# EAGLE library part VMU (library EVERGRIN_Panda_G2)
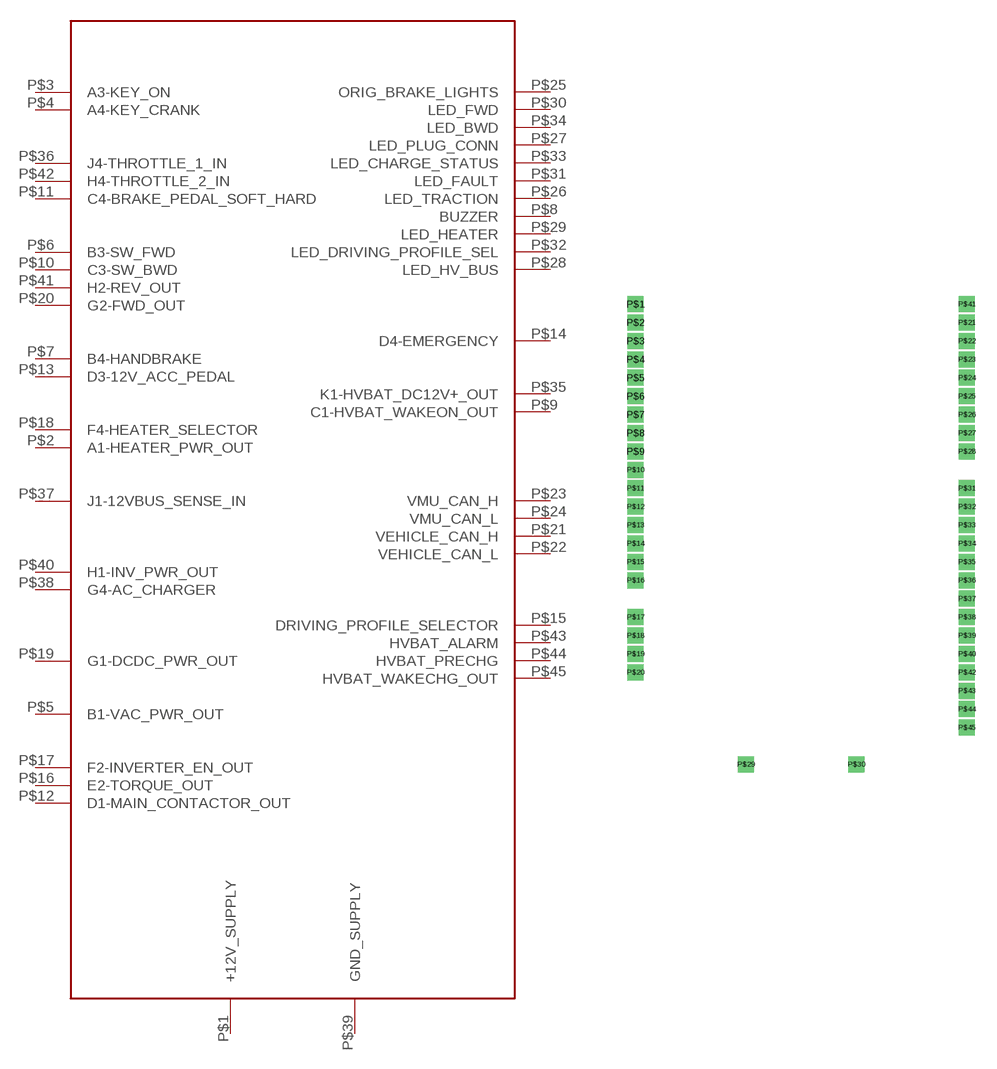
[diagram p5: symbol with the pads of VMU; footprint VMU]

Designator prefix -

## VMU  [VMU]
P$1  +12V_SUPPLY
P$2  A1-HEATER_PWR_OUT  out
P$3  A3-KEY_ON  in
P$4  A4-KEY_CRANK  in
P$5  B1-VAC_PWR_OUT  out
P$6  B3-SW_FWD  in
P$7  B4-HANDBRAKE  in
P$8  BUZZER  out
P$9  C1-HVBAT_WAKEON_OUT  out
P$10  C3-SW_BWD  in
P$11  C4-BRAKE_PEDAL_SOFT_HARD  in
P$12  D1-MAIN_CONTACTOR_OUT  out
P$13  D3-12V_ACC_PEDAL
P$14  D4-EMERGENCY  in
P$15  DRIVING_PROFILE_SELECTOR
P$16  E2-TORQUE_OUT  out
P$17  F2-INVERTER_EN_OUT  out
P$18  F4-HEATER_SELECTOR  in
P$19  G1-DCDC_PWR_OUT  out
P$20  G2-FWD_OUT  in
P$21  VEHICLE_CAN_H
P$22  VEHICLE_CAN_L
P$23  VMU_CAN_H
P$24  VMU_CAN_L
P$25  ORIG_BRAKE_LIGHTS  out
P$26  LED_TRACTION  out
P$27  LED_PLUG_CONN  out
P$28  LED_HV_BUS  out
P$29  LED_HEATER  out
P$30  LED_FWD  out
P$31  LED_FAULT  out
P$32  LED_DRIVING_PROFILE_SEL  out
P$33  LED_CHARGE_STATUS  out
P$34  LED_BWD  out
P$35  K1-HVBAT_DC12V+_OUT  out
P$36  J4-THROTTLE_1_IN  in
P$37  J1-12VBUS_SENSE_IN  in
P$38  G4-AC_CHARGER
P$39  GND_SUPPLY
P$40  H1-INV_PWR_OUT
P$41  H2-REV_OUT  out
P$42  H4-THROTTLE_2_IN  in
P$43  HVBAT_ALARM
P$44  HVBAT_PRECHG
P$45  HVBAT_WAKECHG_OUT

## Footprint VMU (pad centres in mm)
drill 0.6 square: P$1 0,31.75; P$2 0,30.48; P$3 0,29.21; P$4 0,27.94; P$5 0,26.67; P$6 0,25.4; P$7 0,24.13; P$8 0,22.86; P$9 0,21.59; P$10 0,20.32; P$11 0,19.05; P$12 0,17.78; P$13 0,16.51; P$14 0,15.24; P$15 0,13.97; P$16 0,12.7; P$17 0,10.16; P$18 0,8.89; P$19 0,7.62; P$20 0,6.35; P$21 22.86,30.48; P$22 22.86,29.21; P$23 22.86,27.94; P$24 22.86,26.67; P$25 22.86,25.4; P$26 22.86,24.13; P$27 22.86,22.86; P$28 22.86,21.59; P$29 7.62,0; P$30 15.24,0; P$31 22.86,19.05; P$32 22.86,17.78; P$33 22.86,16.51; P$34 22.86,15.24; P$35 22.86,13.97; P$36 22.86,12.7; P$37 22.86,11.43; P$38 22.86,10.16; P$39 22.86,8.89; P$40 22.86,7.62; P$41 22.86,31.75; P$42 22.86,6.35; P$43 22.86,5.08; P$44 22.86,3.81; P$45 22.86,2.54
